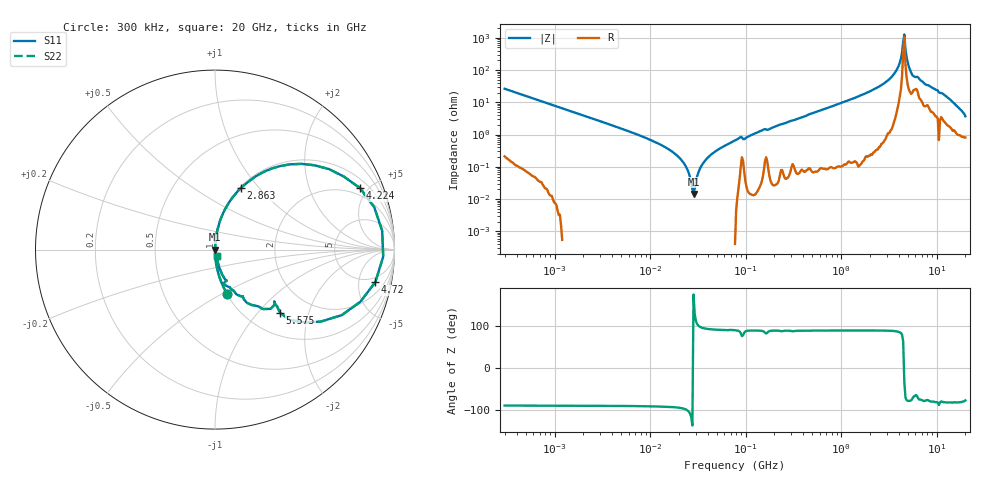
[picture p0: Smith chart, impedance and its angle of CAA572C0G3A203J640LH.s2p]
! S-Parameter Data Generated by TDK Corporation
! Copyright(C) 2022 TDK Corporation.
! All Rights Reserved.
! TDK P/N: CAA572C0G3A203J640LH (Multilayer Ceramic Chip Capacitor)
! Property: C=20nF
! Size(LxWxT): 6x5.6x6.4mm
! Model Type: s2p (Touchstone File Format Version 1.0)
! Frequency: DC=Yes Start=0.3MHz Stop=20000MHz 402points Log-sweep
! Model Generated on Apr. 15, 2022
! Port Assignments:
!  1 ---| |--- 2
! Applicable Conditions:
!  Temperature = 25 degC
!  DC Bias Voltage = 0 V
!  Small Signal Operation
! Terms and conditions regarding TDK Simulation Models
! (1)This simulation model is being provided solely for informational purposes. Please refer to the specifications of the products in terms of detailed characteristics of such products.
! (2)In no event shall TDK Corporation of any of its subsidiaries be liable for any loss or damage arising, directly or indirectly,
!  From any information contained in this simulation model, including, but not limited to loss or damages arising from any inaccuracies, omissions or errors in connection with such information.
! (3)Any and all copyrights on this simulation model are owned by TDK Corporation.
!  Duplication or redistribution of this simulation model without prior written permission from TDK Corporation is prohibited.
! (4)This simulation model is subject to any modification or change without any prior notice.
! (5)Neither TDK Corporation nor any of its subsidiaries shall make any warranty, express or implied,
!  Including but not limited to the correctness, implied warranties of merchantability and fitness for a particular purpose with respect to this simulation models.
! (6)The use of this simulation model shall be deemed to have consented to the terms and conditions hereof.
# Hz S MA R 50
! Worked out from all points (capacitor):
!   401 points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, 300 kHz to 20 GHz, reference 50 ohm
!   read as one part in series: C = 20.1 nF near 317.1 kHz
!   lowest |Z| = 14.5 mohm at 28.51 MHz (marker M1)
!   series resonance near 28.44 MHz, so ESL is about 1.6 nH
!   S11 on the Smith chart (normalised r, x): 300 kHz: 1.00, -0.53; 2.863 GHz: 1.01, +0.80; 4.224 GHz: 1.49, +4.46; 4.72 GHz: 3.83, -8.21; 5.575 GHz: 1.40, -1.32; 20 GHz: 1.02, -0.07
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300000  0.2543 -74.8  0.9651 14.7  0.9651 14.7  0.2543 -74.8
1928084  0.0407 -87.8  0.9993 2.3  0.9993 2.3  0.0407 -87.8
1.239169e7  0.00515 -91.7  1 0.3  1 0.3  0.00515 -91.7
2.159365e7  0.001544 -95.8  1 0.1  1 0.1  0.001544 -95.8
2.413044e7  0.0009233 -99.7  1 0.1  1 0.1  0.0009233 -99.7
2.850518e7  0.0001451 175.1  1 -0.0  1 -0.0  0.0001451 175.1
3.367305e7  0.0009409 97.5  1 -0.1  1 -0.1  0.0009409 97.5
3.868845e7  0.001714 93.4  1 -0.1  1 -0.1  0.001714 93.4
7.964076e7  0.006853 89.2  0.9999 -0.4  0.9999 -0.4  0.006853 89.2
4.978292e8  0.04565 86.5  0.9983 -2.6  0.9983 -2.6  0.04565 86.5
1.470319e9  0.1453 81.1  0.9881 -8.4  0.9881 -8.4  0.1453 81.1
2.863162e9  0.3699 67.3  0.9229 -21.7  0.9229 -21.7  0.3699 67.3
3.199522e9  0.4587 61.5  0.8788 -27.3  0.8788 -27.3  0.4587 61.5
3.886006e9  0.7262 40.3  0.6482 -46.5  0.6482 -46.5  0.7262 40.3
4.2236e9  0.8782 22.9  0.3916 -60.8  0.3916 -60.8  0.8782 22.9
4.464803e9  0.9373 6.4  0.1253 -56.8  0.1253 -56.8  0.9373 6.4
4.719781e9  0.9116 -11.5  0.21 59.5  0.21 59.5  0.9116 -11.5
5.129809e9  0.7122 -34.3  0.5749 44.3  0.5749 44.3  0.7122 -34.3
5.575457e9  0.5045 -44.2  0.7289 28.9  0.7289 28.9  0.5045 -44.2
7.567248e9  0.3219 -59.8  0.8833 18.4  0.8833 18.4  0.3219 -59.8
1.213261e10  0.1609 -72.4  0.9637 9.2  0.9637 9.2  0.1609 -72.4
2e10  0.03646 -75.1  0.9913 2.0  0.9913 2.0  0.03646 -75.1
